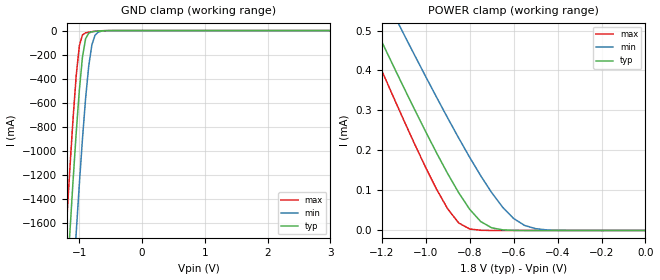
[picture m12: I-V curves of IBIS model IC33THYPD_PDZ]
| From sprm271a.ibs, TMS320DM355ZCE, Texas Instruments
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|   GS50 Cell IC33THYPD
|   Model Cell IC33THYPD_PDZ
[Model]   IC33THYPD_PDZ
Model_type   Input
Polarity   Non-Inverting
Vinl =  0.513
Vinh =  1.323
|Variable   typ   min   max
C_comp   1.003pF   0.997pF   1.008pF
[Temperature Range]   25   125   -40
[Voltage Range]   1.8   1.71   1.89
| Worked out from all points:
|   GND clamp passes 1 mA (typ) near -0.60 V on its own axis
|   POWER clamp passes 1 mA (typ) near -1.65 V on its own axis
[POWER_clamp]
|   voltage   I(typ)   I(min)   I(max)
-3.3V     3.007mA    2.987mA    3.173mA
-1.3V     587.8uA    709uA      526.5uA
-1.25V    529.5uA    654uA      462.8uA
-1.2V     471.6uA    599.3uA    399.6uA
-1.15V    414.2uA    544.9uA    337.1uA
-1.1V     357.4uA    490.9uA    275.5uA
-900mV    141.9uA    281.1uA    53.85uA
-850mV    94.29uA    231.1uA    18.75uA
-750mV    22.33uA    137uA      497.1nA
-650mV    1.547uA    58.07uA    4.65nA
-550mV    45.69nA    12.57uA    282.6pA
0V        421.3pA    11.12nA    177.4pA
[GND_clamp]
|   voltage   I(typ)   I(min)   I(max)
-3.3V     -22.5A     -23.28A    -22.04A
-1.25V    -2.564A    -3.439A    -2.025A
-1.2V     -2.114A    -2.987A    -1.576A
-1.15V    -1.675A    -2.543A    -1.142A
-1.05V    -852.9mA   -1.685A    -376.4mA
-1V       -496.8mA   -1.28A     -126.8mA
-950mV    -219.7mA   -901.6mA   -35.77mA
-900mV    -67.89mA   -564.5mA   -19.05mA
-850mV    -21.23mA   -293.8mA   -13.45mA
-800mV    -10.33mA   -118.7mA   -9.358mA
-650mV    -2.193mA   -5.119mA   -1.521mA
3.3V      421.3pA    69.43nA    157.6pA
